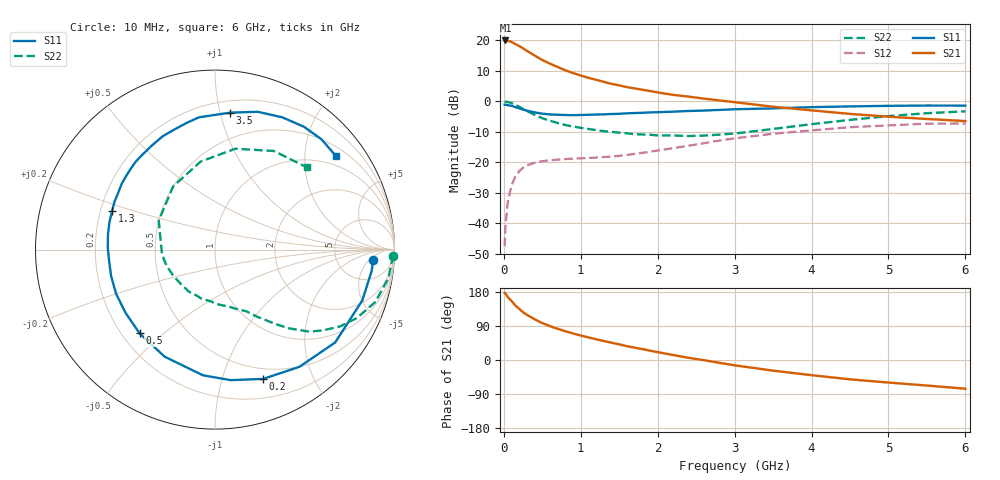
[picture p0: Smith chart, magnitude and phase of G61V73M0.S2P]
! SIEMENS Small Signal Semiconductors
! BFG193
! Si NPN RF Bipolar Junction Transistor in SOT223
! VCE = 1.75 V  IC = 3 mA
! Common Emitter S-Parameters:  August  1996
# GHz  S  MA  R  50
!  f  S11  S21  S12  S22
! GHz  MAG  ANG  MAG  ANG  MAG  ANG  MAG  ANG
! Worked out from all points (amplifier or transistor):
!   36 points, 10 MHz to 6 GHz, reference 50 ohm
!   highest |S21| = 20.0 dB at 20 MHz (marker M1)
!   |S21| within 3 dB of that: start of sweep to 274.9 MHz
!   unconditionally stable (mu >= 1): 1.254 GHz to 2.741 GHz
!   at 250 MHz: K = 0.24, MSG = 19.6 dB, |S12| = -21.8 dB
!   at 1.4 GHz: K = 1.08, MAG = 10.2 dB, |S12| = -18.1 dB
!   at 6 GHz: K = 0.96, MSG = 0.4 dB, |S12| = -7.3 dB
!   S11 on the Smith chart (normalised r, x): 10 MHz: 12, -7; 200 MHz: 0.39, -1.37; 500 MHz: 0.27, -0.42; 1.3 GHz: 0.25, +0.17; 3.5 GHz: 0.29, +1.07; 6 GHz: 0.72, +2.74
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0.01  0.8836 -3.9  9.995 177.3  0.0042 90.0  0.9941 -1.9
0.02  0.8806 -7.9  9.999 175.6  0.0086 84.6  0.9878 -3.7
0.05  0.8683 -19.0  9.873 166.5  0.0218 80.1  0.9786 -9.4
0.1  0.8462 -37.7  9.45 155.8  0.0419 70.7  0.9406 -18.0
0.15  0.8047 -54.3  8.72 143.7  0.0583 61.4  0.878 -25.7
0.2  0.7687 -69.6  8.111 135.0  0.0715 54.6  0.8175 -31.6
0.25  0.7324 -83.2  7.426 126.1  0.0813 48.3  0.7497 -36.9
0.3  0.7035 -95.5  6.746 119.1  0.0888 43.7  0.6969 -41.0
0.4  0.6593 -115.2  5.653 107.6  0.0983 36.5  0.6003 -46.9
0.5  0.6279 -132.0  4.776 97.4  0.1044 31.1  0.5295 -51.2
0.6  0.6103 -144.9  4.159 89.4  0.1082 28.4  0.4795 -54.6
0.7  0.6034 -156.0  3.661 82.3  0.1106 26.2  0.4415 -57.9
0.9  0.5933 -174.0  2.918 70.0  0.115 24.0  0.3862 -63.0
1.1  0.6023 171.9  2.438 59.6  0.1177 24.0  0.3518 -70.0
1.3  0.6124 159.6  2.092 50.1  0.1221 24.8  0.3244 -76.8
1.6  0.6364 144.7  1.713 36.4  0.1323 26.3  0.2994 -90.0
2.2  0.6777 121.5  1.279 13.2  0.1706 26.9  0.2758 -122.1
2.8  0.724 102.4  1.037 -7.4  0.2273 21.0  0.2845 -161.6
3.5  0.7676 83.7  0.817 -28.1  0.2936 6.7  0.3528 152.7
4.5  0.8267 63.1  0.623 -51.1  0.3771 -14.7  0.4972 99.2
5.5  0.8542 46.1  0.514 -67.4  0.4308 -40.7  0.6397 59.2
6  0.8516 37.9  0.475 -75.8  0.4332 -55.2  0.6865 42.0
